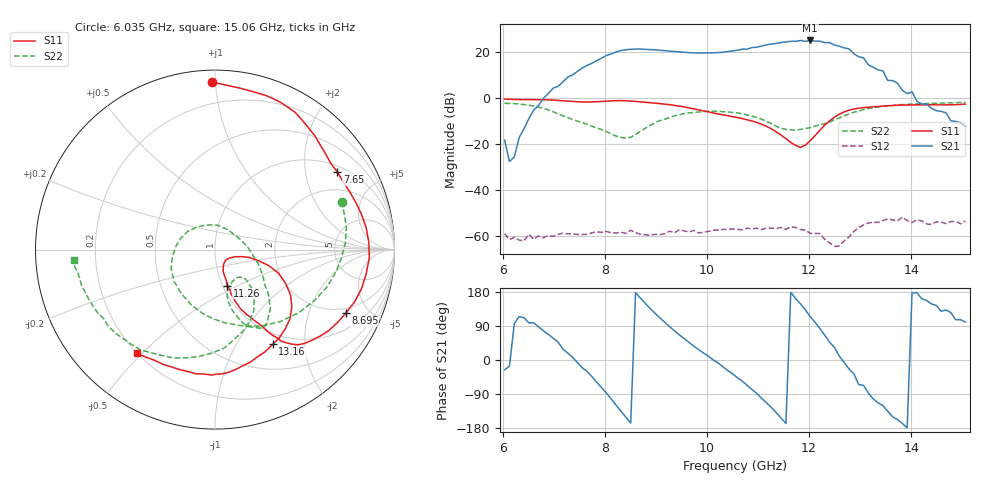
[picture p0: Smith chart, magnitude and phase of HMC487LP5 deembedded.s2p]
!Hittite Microwave Corporation
!20 Alpha Road
!Chelmsford, MA 01824
!Tel: 978-250-3343
!Fax: 978-250-3373
!Device: HMC487LP5, 9-12 GHz, GaAs PHEMT MMIC 2 Watt Power Amplifier in leadless 5x5 mm SMT package
!Misc: Vdd1,2,3,4,5 = +7V, Idd = 1300 mA, Room
# MHZ S MA R 50
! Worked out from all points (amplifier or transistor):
!   96 points, 6.035 GHz to 15.06 GHz, reference 50 ohm
!   highest |S21| = 24.8 dB at 12.02 GHz (marker M1)
!   |S21| within 3 dB of that: 10.93 GHz to 12.66 GHz (1.724 GHz wide, 14.6 % of centre)
!   unconditionally stable (mu >= 1): start of sweep to end of sweep
!   at 7.555 GHz: K = 34.35, MAG = 17.8 dB, |S12| = -59.4 dB
!   at 10.6 GHz: K = 23.00, MAG = 22.3 dB, |S12| = -57.2 dB
!   at 15.06 GHz: K = 178.97, MAG = -5.0 dB, |S12| = -53.5 dB
!   S11 on the Smith chart (normalised r, x): 6.035 GHz: 0.07, +0.98; 7.65 GHz: 1.20, +3.00; 8.695 GHz: 1.72, -3.55; 11.26 GHz: 1.05, -0.44; 13.16 GHz: 0.84, -1.43; 15.06 GHz: 0.20, -0.48
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6035  0.932 90.9  0.12 -26.0  0.001116 -46.3  0.754 20.8
7080  0.87 56.1  1.759 47.7  0.00107 -72.0  0.445 -71.9
7555  0.804 36.6  4.38 -20.5  0.00107 -96.9  0.289 -142.0
7650  0.808 32.4  5.02 -30.0  0.001076 -102.9  0.266 -157.1
8220  0.858 2.6  9.777 -119.6  0.001152 -144.6  0.146 109.7
8505  0.845 -15.0  11.24 -166.5  0.001328 -168.2  0.138 35.6
8695  0.81 -26.0  11.37 163.1  0.001084 -174.1  0.187 2.1
9075  0.74 -43.1  10.69 111.2  0.001063 170.8  0.316 -31.1
9835  0.543 -57.2  9.263 27.2  0.001161 129.5  0.488 -53.0
10595  0.37 -66.0  10.74 -46.8  0.001376 109.2  0.467 -66.6
10880  0.311 -68.7  12.22 -77.9  0.001413 96.4  0.395 -71.5
11260  0.211 -71.5  14.58 -125.5  0.001469 87.5  0.273 -75.5
11640  0.106 -64.2  16.67 178.7  0.001565 80.1  0.2 -58.3
11830  0.083 -43.6  17.4 148.2  0.001371 71.3  0.204 -48.7
12020  0.116 -20.1  17.43 114.4  0.001135 63.2  0.224 -44.1
12115  0.15 -15.1  16.9 99.4  0.001131 63.1  0.242 -44.1
12400  0.311 -16.5  15.71 46.9  0.0007029 67.1  0.296 -46.2
12590  0.436 -25.6  13.13 10.2  0.0006018 96.1  0.362 -52.9
12780  0.533 -36.6  11.48 -23.3  0.0009458 112.1  0.443 -64.0
13160  0.618 -58.6  5.148 -87.1  0.001895 90.8  0.579 -92.3
13635  0.676 -79.8  2.352 -149.9  0.002222 72.3  0.676 -121.8
15060  0.724 -127.0  0.237 100.2  0.002106 26.1  0.79 -175.9
